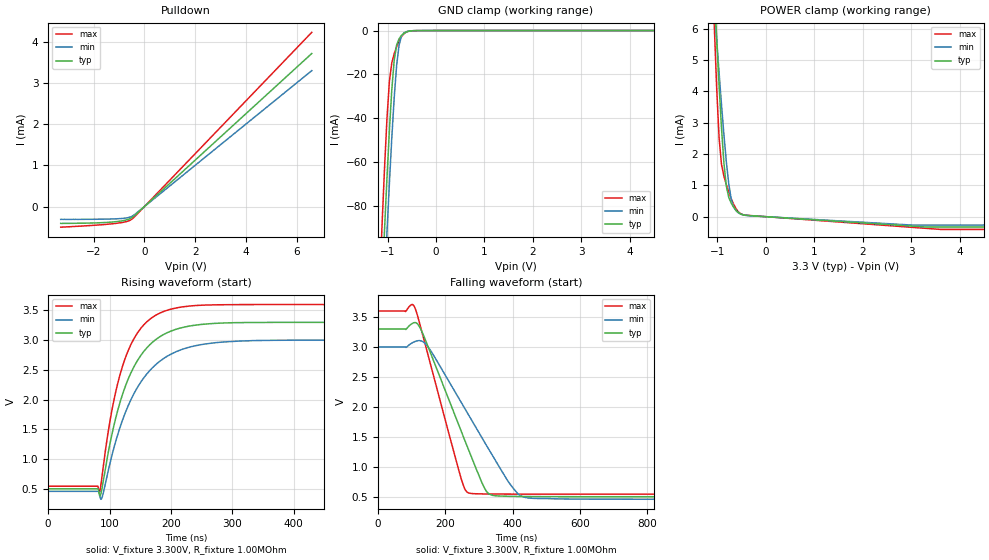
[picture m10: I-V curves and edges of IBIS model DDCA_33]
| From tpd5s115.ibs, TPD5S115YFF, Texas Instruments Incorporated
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[Model]   DDCA_33
Model_type   I/O_open_sink
Vinl = 800.000mV
Vinh = 2.000V
Vmeas = 1.500V
Cref = 15pF
Rref = 1000000
Vref = 0V
|   typ   min   max
|3-state
C_comp   1.1397pF   1.1025pF   1.2215pF
|pulldown
|C_comp   1.1949pF   1.1694pF   1.2499pF
[Voltage Range]   3.300V   3.000V   3.600V
|Junction temperature
[Temperature Range]   40.0   100.0   -40.0
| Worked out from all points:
|   slope of the pulldown table from 0 to 0.495 V, typ, clamps not added: 1.78 kohm
|   GND clamp passes 1 mA (typ) near -0.64 V on its own axis
|   POWER clamp passes 1 mA (typ) near -0.81 V on its own axis
|   falling waveform, V_fixture 3.300V, R_fixture 1.00MOhm: 20-80 % time 118ns typ, 160ns min, 86.9ns max; typ from 3.3 V to 0.5 V
|   rising waveform, V_fixture 3.300V, R_fixture 1.00MOhm: 20-80 % time 53.8ns typ, 64.2ns min, 44.5ns max; typ from 0.5 V to 3.3 V
|ambient temperature   25   85   -40|
[Pulldown]
|   Voltage   I(typ)   I(min)   I(max)
-3.3V     -408uA     -310uA     -499uA
-1.26V    -374.2uA   -299.8uA   -416.6uA
-713.1mV  -323.4uA   -276.2uA   -364.4uA
-464.3mV  -254.2uA   -225.1uA   -290.7uA
6.6V      3.714mA    3.298mA    4.228mA
[GND Clamp]
|   Voltage   I(typ)   I(min)   I(max)
-3.3V     -2.285A    -2.051A    -2.629A
-1.161V   -140.4mA   -164mA     -114.1mA
-1.111V   -115.1mA   -139.3mA   -87.51mA
-1.061V   -90.52mA   -115.3mA   -62.41mA
-1.012V   -67.11mA   -91.95mA   -40mA
-961.8mV  -45.48mA   -69.67mA   -23.17mA
-912.1mV  -26.88mA   -48.92mA   -14.71mA
-862.3mV  -13.5mA    -30.52mA   -10.56mA
-812.6mV  -6.659mA   -15.92mA   -7.423mA
-713.1mV  -2.253mA   -2.629mA   -2.864mA
-613.6mV  -659.8uA   -538.9uA   -689.6uA
6.6V      0A         0A         0A
[POWER Clamp]
|   Voltage   I(typ)   I(min)   I(max)
-3.3V     65.62mA    7.928mA    101.1mA
-1.061V   7.235mA    6.729mA    6.104mA
-1.012V   5.665mA    5.643mA    4.086mA
-961.8mV  4.175mA    4.586mA    2.508mA
-912.1mV  2.82mA     3.569mA    1.665mA
-862.3mV  1.704mA    2.613mA    1.292mA
-812.6mV  972uA      1.753mA    1.026mA
-713.1mV  434.4uA    569.2uA    581.2uA
-613.6mV  207.3uA    190uA      257uA
-514.1mV  85.98uA    78.49uA    91.47uA
3.615V    -330uA     -268uA     -407.5uA
6.6V      -330uA     -268uA     -407.5uA
[Ramp]
R_load = 1.00MOhm
|   typ   min   max
dV/dt_r   1.680V/53.773ns   1.526V/64.160ns   1.834V/44.463ns
dV/dt_f   1.680V/117.747ns   1.526V/159.869ns   1.834V/86.893ns
[Falling Waveform]
V_fixture = 3.300V
V_fixture_min = 3.000V
V_fixture_max = 3.600V
R_fixture = 1.00MOhm
|   Time   V(typ)   V(min)   V(max)
0s        3.3V       3V         3.6V
83ns      3.292V     2.994V     3.594V
109ns     3.407V     3.088V     3.667V
151ns     2.977V     2.986V     2.821V
247ns     1.6V       2.078V     805.5mV
271ns     1.26V      1.848V     560.6mV
329ns     552.5mV    1.295V     545.6mV
402ns     505.5mV    641.1mV    543.8mV
445ns     503mV      480.2mV    543.4mV
1.914us   499.8mV    456.7mV    542.7mV
[Rising Waveform]
V_fixture = 3.300V
V_fixture_min = 3.000V
V_fixture_max = 3.600V
R_fixture = 1.00MOhm
|   Time   V(typ)   V(min)   V(max)
0s        499.8mV    456.7mV    542.7mV
81ns      499.8mV    456.7mV    542.7mV
84ns      379.4mV    395.8mV    445.3mV
88ns      520.2mV    358mV      727.9mV
107ns     1.558V     1.184V     1.984V
132ns     2.384V     1.935V     2.862V
165ns     2.917V     2.483V     3.346V
216ns     3.205V     2.837V     3.556V
368ns     3.299V     2.998V     3.6V
1.914us   3.3V       3V         3.6V
